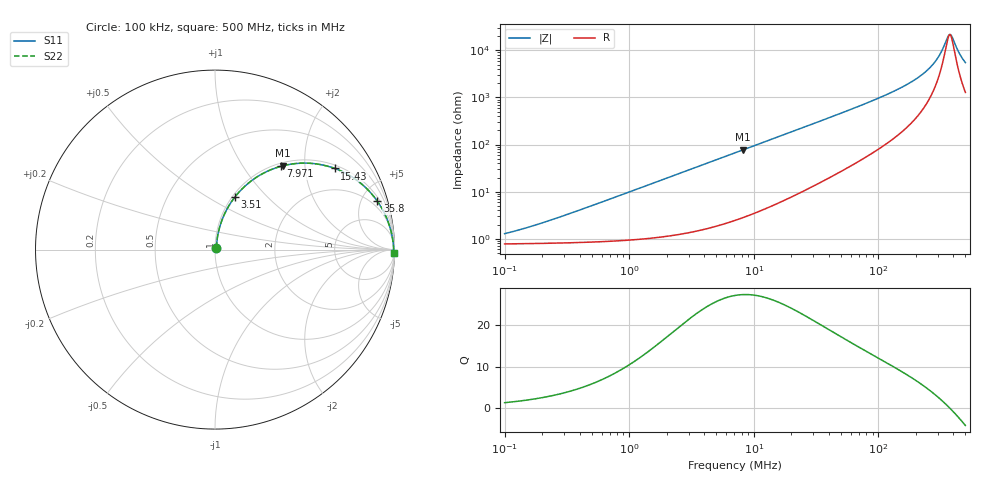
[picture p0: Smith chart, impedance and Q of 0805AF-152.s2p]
# MHz  S  MA  R  50
!Freq  MagS11  AngS11  MagS21  AngS21  MagS12  AngS12  MagS22  AngS22
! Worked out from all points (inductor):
!   801 points, 100 kHz to 500 MHz, reference 50 ohm
!   read as one part in series: L = 1.6 uH near 242.1 kHz
!   highest Q = 27.4 at 8.23 MHz (marker M1), where L = 1.5 uH
!   self-resonance near 373 MHz
!   S11 on the Smith chart (normalised r, x): 100 kHz: 1.02, +0.02; 3.51 MHz: 1.03, +0.67; 7.971 MHz: 1.05, +1.50; 15.43 MHz: 1.11, +2.87; 35.8 MHz: 1.33, +6.60; 500 MHz: open
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0.1  0.01279 52.1  0.9922 -0.6  0.9922 -0.6  0.01279 52.1
0.179664  0.01973 65.3  0.9919 -1.0  0.9919 -1.0  0.01973 65.3
0.4168304  0.04207 76.2  0.9908 -2.4  0.9908 -2.4  0.04207 76.2
1.719065  0.1634 76.9  0.9761 -9.4  0.9761 -9.4  0.1634 76.9
3.509716  0.3149 69.2  0.9355 -18.3  0.9355 -18.3  0.3149 69.2
7.089654  0.5477 54.7  0.8168 -33.2  0.8168 -33.2  0.5477 54.7
7.971081  0.5908 51.7  0.7855 -36.2  0.7855 -36.2  0.5908 51.7
8.229945  0.6025 50.9  0.7764 -37.0  0.7764 -37.0  0.6025 50.9
11.20901  0.7114 42.6  0.677 -45.3  0.677 -45.3  0.7114 42.6
15.42994  0.8064 34.1  0.5608 -53.7  0.5608 -53.7  0.8064 34.1
29.55184  0.925 19.8  0.3389 -67.5  0.3389 -67.5  0.925 19.8
35.79831  0.944 16.6  0.2858 -70.5  0.2858 -70.5  0.944 16.6
121.8757  0.989 4.7  0.08151 -80.0  0.08151 -80.0  0.989 4.7
186.6293  0.9928 2.6  0.04548 -79.6  0.04548 -79.6  0.9928 2.6
251.4916  0.9943 1.4  0.02519 -76.2  0.02519 -76.2  0.9943 1.4
301.4221  0.9949 0.8  0.01415 -68.6  0.01415 -68.6  0.9949 0.8
324.7589  0.9951 0.5  0.00995 -60.4  0.00995 -60.4  0.9951 0.5
357.4375  0.9953 0.2  0.005491 -31.7  0.005491 -31.7  0.9953 0.2
372.9979  0.9954 0.0  0.004606 -4.1  0.004606 -4.1  0.9954 0.0
389.2357  0.9955 -0.1  0.005053 26.2  0.005053 26.2  0.9955 -0.1
451.8398  0.9956 -0.6  0.01212 68.4  0.01212 68.4  0.9956 -0.6
500  0.9956 -1.0  0.01814 75.5  0.01814 75.5  0.9956 -1.0
